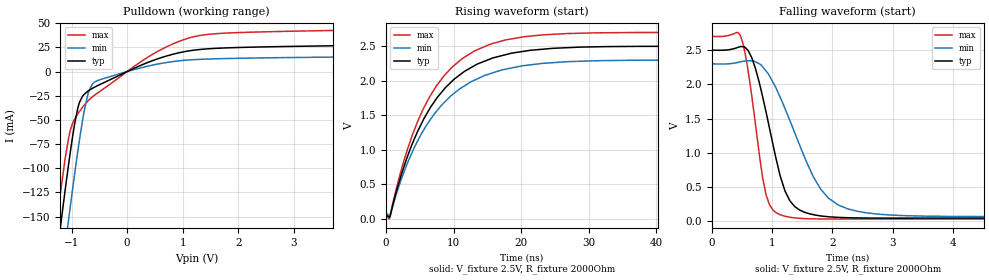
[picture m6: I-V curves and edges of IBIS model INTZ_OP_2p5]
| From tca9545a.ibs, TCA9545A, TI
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|   Model
[Model]   INTZ_OP_2p5
Model_type   Open_drain
Polarity   Non-Inverting
Vmeas = 1.25
Vref = 2.5
Cref = 1pF
Rref = 2000
|   typ   min   max
C_comp   1.601pF   1.487pF   1.862pF
[Voltage Range]   2.5   2.3   2.7
[Temperature Range]   27   125   -40
[Pullup Reference]   2.5   2.3   2.7
[Pulldown Reference]   -0   -0   -0
[Power Clamp Reference]   2.5   2.3   2.7
[GND Clamp Reference]   -0   -0   -0
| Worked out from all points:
|   slope of the pulldown table from 0 to 0.375 V, typ, clamps not added: 39.6 ohm
|   falling waveform, V_fixture 2.5V, R_fixture 2000Ohm: 20-80 % time 387ps typ, 661ps min, 251ps max; typ from 2.5 V to 0.044 V
|   rising waveform, V_fixture 2.5V, R_fixture 2000Ohm: 20-80 % time 7.97ns typ, 8.46ns min, 7.6ns max; typ from 0.044 V to 2.5 V
[Pulldown]
|   Voltage   I(typ)   I(min)   I(max)
-2.5V     -787.4mA   -845.7mA   -751.3mA
-1.27V    -192.5mA   -252.3mA   -156.2mA
-1.225V   -171.8mA   -231.3mA   -136.1mA
-1.105V   -118mA     -176.4mA   -86.18mA
-1.045V   -92.45mA   -149.5mA   -66.36mA
-940mV    -52.67mA   -104mA     -48.68mA
-865mV    -33.18mA   -73.5mA    -41.9mA
-700mV    -20.01mA   -22.06mA   -30.05mA
-520mV    -14.24mA   -9.04mA    -21.66mA
492.5mV   12mA       7.084mA    18.95mA
1.265V    22.56mA    12.5mA     36.8mA
4.992V    27.7mA     15.68mA    43.84mA
[Ramp]
R_load = 2000
|   typ   min   max
dV/dt_r   1.4733/7.97116e-09   1.33949/8.46169e-09   1.60149/7.60719e-09
dV/dt_f   1.47332/3.86759e-10   1.33951/6.61447e-10   1.60151/2.5124e-10
[Falling Waveform]
V_fixture = 2.5V
V_fixture_min = 2.3V
V_fixture_max = 2.7V
R_fixture = 2000Ohm
C_fixture = 0F
|   Time   V(typ)   V(min)   V(max)
0s        2.5V       2.3V       2.7V
511.6ps   2.55V      2.333V     2.62V
726.7ps   2.228V     2.328V     1.41V
842.8ps   1.826V     2.257V     644.6mV
957ps     1.363V     2.124V     242.4mV
1.294ns   298.8mV    1.472V     57.69mV
1.668ns   98.24mV    677.6mV    33.49mV
2.251ns   50.57mV    179.8mV    30.93mV
3.975ns   44.67mV    69.22mV    30.93mV
100ns     44.47mV    67.48mV    30.82mV
[Rising Waveform]
V_fixture = 2.5V
V_fixture_min = 2.3V
V_fixture_max = 2.7V
R_fixture = 2000Ohm
C_fixture = 0F
|   Time   V(typ)   V(min)   V(max)
0s        44.47mV    67.48mV    30.82mV
511.6ps   24.57mV    53.46mV    1.491mV
2.052ns   569mV      514.4mV    635.3mV
3.862ns   1.082V     964.3mV    1.205V
5.527ns   1.437V     1.28V      1.597V
7.372ns   1.729V     1.547V     1.915V
11.33ns   2.117V     1.91V      2.326V
17.72ns   2.38V      2.17V      2.594V
31.15ns   2.493V     2.292V     2.696V
100ns     2.5V       2.3V       2.7V
